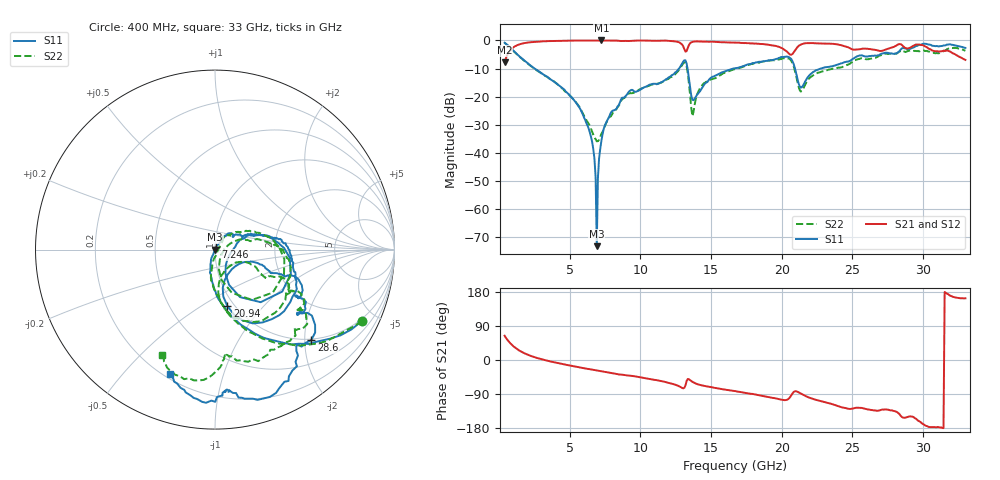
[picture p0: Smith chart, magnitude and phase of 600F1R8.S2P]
!  American Technical Ceramics  Date:  11/23/05
!  One Norden Lane
!  Huntington Station,  NY.  11746-2102
!  Tel:  (631) 622-4700  Fax:  (631) 622-4748
!  Part Number  600F1R8  Mounting Orientation: Horizontal
!  Description: Ultra Low ESR Microwave capacitors
!  Application: Coupling, Bypass, Tuning, DC Block
!  Filters, Matching
# GHZ S DB R 50
! Freq  |S11|  S11 Ph  |S21|  S21 Ph  |S12|  S12 Ph  |S22|  S22 Ph
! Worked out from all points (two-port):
!   401 points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, 400 MHz to 33 GHz, reference 50 ohm
!   highest |S21| = 0.00 dB at 7.246 GHz (marker M1); lowest = -7.8 dB at 400 MHz (marker M2)
!   |S21| within 3 dB of the highest: 899.5 MHz to 13.11 GHz (12.21 GHz wide, 174 % of centre); 13.33 GHz to 20.11 GHz (6.772 GHz wide, 40.5 % of centre)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
!   lowest |S11| = -73.3 dB at 6.92 GHz (marker M3), VSWR 1.00, Z = 50 - j0.0179 ohm
!   |S11| at or under -10 dB: 2.516 GHz to 12.74 GHz (10.22 GHz wide, 134 % of centre); 13.34 GHz to 16.61 GHz (3.267 GHz wide, 21.8 % of centre); 20.94 GHz to 22.8 GHz (1.854 GHz wide, 8.48 % of centre)
!   |S22| runs from -36.0 to -0.8 dB; largest |S21 - S12| = 0.015
!   S11 on the Smith chart (normalised r, x): 400 MHz: 0.90, -4.18; 7.246 GHz: 1.01, +0.03; 20.94 GHz: 0.93, -0.65; 28.6 GHz: 0.98, -2.15; 33 GHz: 0.22, -0.68
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0.4  -0.81 -25.8  -7.79 64.0  -7.79 63.9  -0.80 -26.1
2.112  -8.47 -76.4  -0.69 12.9  -0.70 12.6  -8.51 -77.5
5.861  -25.59 -112.7  -0.01 -20.6  -0.01 -20.6  -25.31 -97.7
6.513  -34.40 -111.0  -0.02 -24.9  -0.02 -24.9  -31.49 -72.9
6.92  -73.35 -123.5  0.00 -27.5  0.00 -27.6  -35.96 -29.7
7.083  -42.11 70.2  -0.01 -28.6  -0.01 -28.7  -35.43 -2.0
7.246  -35.83 68.6  0.00 -29.8  -0.01 -29.8  -33.32 15.1
7.735  -27.84 57.0  0.00 -33.0  -0.01 -33.0  -28.00 37.9
8.795  -20.45 51.2  -0.16 -39.2  -0.15 -39.1  -20.66 49.0
11.321  -15.28 25.4  -0.09 -54.2  -0.09 -54.1  -15.32 34.5
13.114  -7.07 -17.6  -3.07 -73.5  -3.03 -73.1  -7.79 -19.5
13.766  -21.30 -21.2  -0.41 -59.2  -0.41 -59.2  -25.41 2.6
14.5  -15.88 21.4  -0.41 -67.9  -0.41 -67.9  -15.26 18.7
16.7  -9.93 12.5  -0.75 -82.2  -0.75 -81.9  -10.18 6.6
19.96  -5.92 -25.7  -2.56 -104.6  -2.63 -104.3  -6.66 -30.4
20.938  -9.88 -77.7  -3.59 -82.6  -3.64 -82.8  -10.80 -84.1
21.346  -16.82 -49.9  -1.50 -88.2  -1.52 -88.1  -18.21 -54.3
22.161  -11.56 -18.3  -0.93 -102.0  -0.94 -102.1  -12.67 -22.7
27.621  -4.66 -37.3  -2.82 -132.0  -2.78 -131.6  -4.69 -34.7
28.599  -2.66 -43.3  -2.04 -152.1  -2.06 -151.8  -3.86 -43.7
30.229  -1.21 -74.2  -2.30 -174.0  -2.34 -174.3  -3.72 -73.5
33  -2.65 -110.1  -6.93 162.8  -6.87 163.0  -3.68 -116.6
